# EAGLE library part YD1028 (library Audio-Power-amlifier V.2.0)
18W CAR RADIO POWER AMPLIFIER
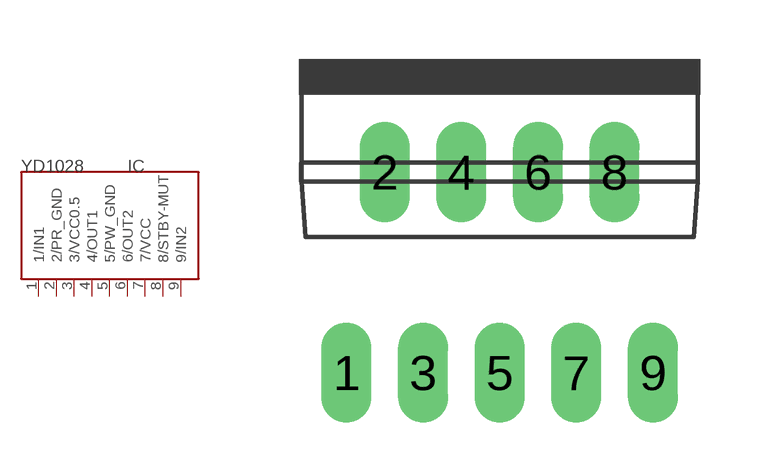
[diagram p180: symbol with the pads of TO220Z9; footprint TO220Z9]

Designator prefix IC

## YD1028  [TO220Z9]
1  1/IN1  in
2  2/PR_GND  pwr
3  3/VCC0.5  pwr
4  4/OUT1  out
5  5/PW_GND  pwr
6  6/OUT2  out
7  7/VCC  pwr
8  8/STBY-MUT  in
9  9/IN2  in

## Footprint TO220Z9 (pad centres in mm)
9-lead single in-line (TO220Z9) plastic power package
drill 0.5 pad 1.27 long: 1 -3.88,-5.08; 2 -2.91,0; 3 -1.94,-5.08; 4 -0.97,0; 5 0,-5.08; 6 0.97,0; 7 1.94,-5.08; 8 2.91,0; 9 3.88,-5.08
